|   TEXAS INSTRUMENTS INCORPORATED
|   Standard Linear and Logic
|   IBIS Model of SN74LVTH16952
|   3.3V ABT 16 BIT  Registered Transceiver with 3-STATE OUTPUTS
|   TSSOP 56 PIN PACKAGE (DGG)
|   SSOP 56 PIN PACKAGE (DL)
[IBIS Ver]   2.1
[Comment char]   |_char
[File Name]   sn74lvth16952.ibs
[File Rev]   1.0
[Date]   06-08-2000
[Source]   Data created from HSPICE simulations at TI ,SLL.
[Notes]   The following is an IBIS list for LVTH16952
   - All test data contained in this file are derived from hspice
   (tm) simulations.
   - This file may be incomplete or may not be fully compliant
   with the IBIS specification. It will be replaced with a
   version that is IBIS Revision 3.2 compliant and is complete
   and accurate. Please email all questions and comments to
   sllibis@ti.com.
|   -For Questions or Comments please mailto:sllibis@ti.com
|  [Disclaimer]
|*   Property of Texas Instruments Incorporated.  Unauthorized   *
|*   reproduction and/or distribution is strictly prohibited.   *
|*   This product is protected under copyright law.   *
|*   Created 1995, (C) Copyright 1995, Texas Instruments Inc.,   *
|*   All Rights Reserved   *
|*   UNLESS THERE IS A SIGNED, WRITTEN AGREEMENT TO THE   *
|*   CONTRARY, TEXAS INSTRUMENTS ("TI") IS PROVIDING THE SPICE   *
|*   MODELS "AS IS" AND WITHOUT ANY WARRANTY, EXPRESSED OR   *
|*   IMPLIED.  TI assumes no liability for:   *
|*   1) the accuracy of the IBIS models provided to your   *
|*   company;   *
|*   2) the proper functioning of these IBIS models in your   *
|*   design or for any resulting applications; or   *
|*   3) infringement of patents, copyrights or intellectual   *
|*   property rights resulting from your use of these   *
|*   IBIS models.   *
|*   TI provides IBIS Models as a service to our customers.   *
|*   You and your company shall not distribute, sell or give   *
|*   these models to anyone else without prior written   *
|*   permission from TI.   *
|*   TI reserves the right to make changes to our products or   *
|*   to discontinue any semiconductor product or service   *
|*   without notice, and advises our customers to obtain the   *
|*   latest version of relevant information to verify, before   *
|*   placing orders, that the information being relied on is   *
|*   current.   *
|*   Please be aware that your receipt and use of the IBIS   *
|*   information provided shall serve as acceptance of these   *
|*   terms and conditions.  If you do not accept these terms,   *
|*   you should return or destroy the IBIS models and any   *
|*   other accompanying information immediately.   *
[Component]   LVTH16952_DGG
[manufacturer]   Texas Instruments, Inc.
[Package]
|   typ   min   max
   R_pkg   0.045   0.035   0.062
   L_pkg   3.324nH   2.403nH   5.094nH
   C_pkg   0.564pF   0.341pF   0.914nH
[Pin]   signal_name   model_name   R_pin   L_pin   C_pin
1   1NOEAB   NOE   0.062   5.094nH   0.856pF
2   1CLKAB   CLK   0.061   4.621nH   0.902pF
3   1NCLKENAB   CLKEN   0.06   4.316nH   0.802pF
4   GND   GND   0.059   3.968nH   0.698pF
5   1A1   LVTH16952_IO   0.057   3.716nH   0.649pF
6   1A2   LVTH16952_IO   0.042   3.517nH   0.652pF
7   VCC   POWER   0.041   3.16nH   0.57pF
8   1A3   LVTH16952_IO   0.039   2.981nH   0.482pF
9   1A4   LVTH16952_IO   0.039   2.809nH   0.447pF
10   1A5   LVTH16952_IO   0.038   2.715nH   0.409pF
11   GND   GND   0.041   2.675nH   0.391pF
12   1A6   LVTH16952_IO   0.039   2.536nH   0.366pF
13   1A7   LVTH16952_IO   0.039   2.457nH   0.348pF
14   1A8   LVTH16952_IO   0.038   2.411nH   0.353pF
15   2A1   LVTH16952_IO   0.039   2.456nH   0.355pF
16   2A2   LVTH16952_IO   0.039   2.471nH   0.349pF
17   2A3   LVTH16952_IO   0.04   2.58nH   0.37pF
18   GND   GND   0.038   2.651nH   0.389pF
19   2A4   LVTH16952_IO   0.038   2.739nH   0.411pF
20   2A5   LVTH16952_IO   0.039   2.838nH   0.449pF
21   2A6   LVTH16952_IO   0.038   2.988nH   0.484pF
22   VCC   POWER   0.038   3.105nH   0.564pF
23   2A7   LVTH16952_IO   0.04   3.427nH   0.638pF
24   2A8   LVTH16952_IO   0.056   3.654nH   0.641pF
25   GND   GND   0.057   3.932nH   0.7pF
26   2NCLKENAB  CLKEN   0.058   4.257nH   0.806pF
27   2CLKAB   CLK   0.057   4.58nH   0.914pF
28   2NOEAB   NOE   0.059   5.038nH   0.861pF
29   2NOEBA   NOE   0.06   5.058nH   0.858pF
30   2CLKBA   CLK   0.056   4.543nH   0.904pF
31   2NCLKENBA  CLKEN   0.057   4.24nH   0.803pF
32   GND   GND   0.057   3.929nH   0.7pF
33   2B8   LVTH16952_IO   0.056   3.616nH   0.637pF
34   2B7   LVTH16952_IO   0.037   3.368nH   0.64pF
35   VCC   POWER   0.036   3.024nH   0.563pF
36   2B6   LVTH16952_IO   0.035   2.876nH   0.474pF
37   2B5   LVTH16952_IO   0.035   2.745nH   0.444pF
38   2B4   LVTH16952_IO   0.037   2.683nH   0.405pF
39   GND   GND   0.038   2.603nH   0.382pF
40   2B3   LVTH16952_IO   0.038   2.51nH   0.362pF
41   2B2   LVTH16952_IO   0.036   2.412nH   0.341pF
42   2B1   LVTH16952_IO   0.038   2.416nH   0.349pF
43   1B8   LVTH16952_IO   0.037   2.403nH   0.349pF
44   1B7   LVTH16952_IO   0.037   2.429nH   0.341pF
45   1B6   LVTH16952_IO   0.036   2.482nH   0.358pF
46   GND   GND   0.037   2.615nH   0.381pF
47   1B5   LVTH16952_IO   0.035   2.669nH   0.402pF
48   1B4   LVTH16952_IO   0.036   2.763nH   0.442pF
49   1B3   LVTH16952_IO   0.036   2.942nH   0.478pF
50   VCC   POWER   0.035   3.053nH   0.564pF
51   1B2   LVTH16952_IO   0.036   3.409nH   0.641pF
52   1B1   LVTH16952_IO   0.058   3.698nH   0.641pF
53   GND   GND   0.059   3.975nH   0.697pF
54   1NCLKENBA  CLKEN   0.061   4.327nH   0.802pF
55   1CLKBA   CLK   0.061   4.624nH   0.905pF
56   1NOEBA   NOE   0.06   5.063nH   0.858pF
[Component]   LVTH16952_DL
[manufacturer]   Texas Instruments Inc.
[Package]
|   typ   min   max
R_pkg   0.055   0.048   0.067
L_pkg   6.539nH   4.802nH   9.746nH
C_pkg   .857pF   0.5pF   1.351pF
[Pin]   signal_name   model_name   R_pin   L_pin   C_pin
1   1NOEAB   NOE   0.064   9.646nH   1.202pF
2   1CLKAB   CLK   0.059   8.723nH   1.348pF
3   1NCLKENAB   CLKEN   0.059   8.139nH   1.223pF
4   GND   GND   0.056   7.554nH   1.088pF
5   1A1   LVTH16952_IO   0.054   6.991nH   0.966pF
6   1A2   LVTH16952_IO   0.053   6.659nH   0.973pF
7   VCC   POWER   0.055   6.321nH   0.905pF
8   1A3   LVTH16952_IO   0.055   5.942nH   0.713pF
9   1A4   LVTH16952_IO   0.057   5.767nH   0.678pF
10   1A5   LVTH16952_IO   0.054   5.459nH   0.631pF
11   GND   GND   0.051   5.224nH   0.638pF
12   1A6   LVTH16952_IO   0.048   5.088nH   0.601pF
13   1A7   LVTH16952_IO   0.05   5.021nH   0.518pF
14   1A8   LVTH16952_IO   0.051   4.802nH   0.5pF
15   2A1   LVTH16952_IO   0.051   4.803nH   0.5pF
16   2A2   LVTH16952_IO   0.05   5.021nH   0.518pF
17   2A3   LVTH16952_IO   0.048   5.088nH   0.601pF
18   GND   GND   0.051   5.224nH   0.638pF
19   2A4   LVTH16952_IO   0.054   5.459nH   0.631pF
20   2A5   LVTH16952_IO   0.057   5.768nH   0.677pF
21   2A6   LVTH16952_IO   0.055   5.942nH   0.715pF
22   VCC   POWER   0.055   6.321nH   0.907pF
23   2A7   LVTH16952_IO   0.053   6.659nH   0.972pF
24   2A8   LVTH16952_IO   0.054   6.991nH   0.966pF
25   GND   GND   0.056   7.554nH   1.087pF
26   2NCLKENAB   CLKEN   0.059   8.139nH   1.223pF
27   2CLKAB   CLK   0.059   8.727nH   1.351pF
28   2NOEAB   NOE   0.067   9.746nH   1.21pF
29   2NOEBA   NOE   0.063   9.63nH   1.203pF
30   2CLKBA   CLK   0.06   8.751nH   1.349pF
31   2NCLKENBA   CLKEN   0.06   8.184nH   1.224pF
32   GND   GND   0.056   7.543nH   1.087pF
33   2B8   LVTH16952_IO   0.054   7.005nH   0.969pF
34   2B7   LVTH16952_IO   0.056   6.714nH   0.975pF
35   VCC   POWER   0.058   6.384nH   0.909pF
36   2B6   LVTH16952_IO   0.057   5.976nH   0.717pF
37   2B5   LVTH16952_IO   0.057   5.743nH   0.677pF
38   2B4   LVTH16952_IO   0.055   5.469nH   0.631pF
39   GND   GND   0.055   5.328nH   0.644pF
40   2B3   LVTH16952_IO   0.052   5.189nH   0.606pF
41   2B2   LVTH16952_IO   0.052   5.053nH   0.519pF
42   2B1   LVTH16952_IO   0.052   4.825nH   0.502pF
43   1B8   LVTH16952_IO   0.054   4.896nH   0.506pF
44   1B7   LVTH16952_IO   0.052   5.093nH   0.521pF
45   1B6   LVTH16952_IO   0.051   5.179nH   0.608pF
46   GND   GND   0.054   5.314nH   0.645pF
47   1B5   LVTH16952_IO   0.055   5.511nH   0.632pF
48   1B4   LVTH16952_IO   0.057   5.77nH   0.677pF
49   1B3   LVTH16952_IO   0.055   5.956nH   0.716pF
50   VCC   POWER   0.055   6.32nH   0.905pF
51   1B2   LVTH16952_IO   0.052   6.621nH   0.968pF
52   1B1   LVTH16952_IO   0.053   6.974nH   0.966pF
53   GND   GND   0.057   7.571nH   1.089pF
54   1NCLKENBA   CLKEN   0.057   8.097nH   1.219pF
55   1CLKBA   CLK   0.059   8.723nH   1.349pF
56   1NOEBA   NOE   0.061   9.56nH   1.199pF
| Models and submodels in the file (4): LVTH16952_IO (I/O), CLK (Input), CLKEN (Input), NOE (Input)
